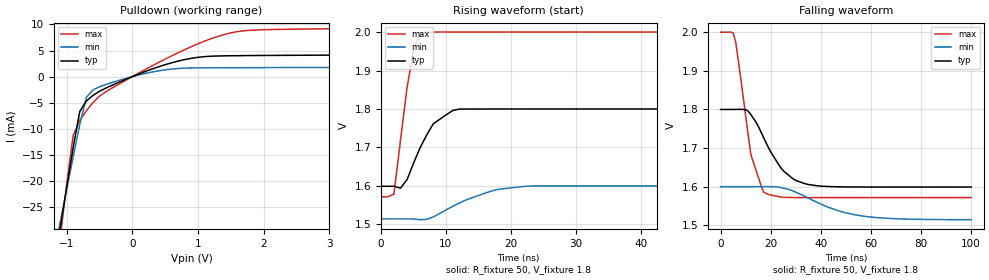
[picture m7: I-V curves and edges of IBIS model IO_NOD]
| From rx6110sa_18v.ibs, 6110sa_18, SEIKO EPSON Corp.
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[Model]   IO_NOD
Model_type Open_drain
Enable Active-Low
Polarity Non-Inverting
Vref=1.8
Vmeas=0.9
Rref=5000
C_comp   2.5p   2p   3p
[Temperature Range] 25   85   -40
[Voltage Range]   1.8   1.6   2.0
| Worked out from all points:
|   slope of the pulldown table from 0 to 0.27 V, typ, clamps not added: 206 ohm
|   falling waveform, R_fixture 50, V_fixture 1.8: 20-80 % time 10.6ns typ, 19.5ns min, 6.06ns max; typ from 1.8 V to 1.6 V
|   rising waveform, R_fixture 50, V_fixture 1.8: 20-80 % time 3.44ns typ, 6.96ns min, 2.06ns max; typ from 1.6 V to 1.8 V
[Pulldown]
-1.8V     -86.42mA   -77.23mA   -105.3mA
-1.1V     -29.16mA   -28.04mA   -31.08mA
-1V       -21.31mA   -21.63mA   -20.71mA
-900mV    -13.53mA   -15.35mA   -11.23mA
-800mV    -6.683mA   -9.177mA   -8.363mA
-700mV    -4.673mA   -3.993mA   -6.555mA
-500mV    -2.814mA   -1.945mA   -3.752mA
100mV     507uA      322.3uA    694.9uA
600mV     2.655mA    1.451mA    3.99mA
1.4V      3.983mA    1.706mA    8.072mA
1.9V      4.05mA     1.725mA    8.952mA
3.6V      4.155mA    1.772mA    9.24mA
[Falling Waveform]
R_fixture=50
V_fixture=1.8
V_fixture_min=1.6
V_fixture_max=2.0
0s        1.8V       1.6V       2V
5.051ns   1.8V       1.6V       1.998V
6.061ns   1.8V       1.6V       1.974V
10.1ns    1.799V     1.6V       1.78V
12.12ns   1.786V     1.6V       1.683V
17.17ns   1.727V     1.6V       1.586V
24.24ns   1.647V     1.597V     1.573V
34.34ns   1.607V     1.573V     1.572V
57.58ns   1.599V     1.523V     1.572V
100ns     1.599V     1.515V     1.572V
[Rising Waveform]
R_fixture=50
V_fixture=1.8
V_fixture_min=1.6
V_fixture_max=2.0
0s        1.599V     1.514V     1.572V
2.02ns    1.599V     1.514V     1.578V
3.03ns    1.594V     1.514V     1.718V
4.04ns    1.616V     1.514V     1.855V
5.051ns   1.659V     1.514V     1.953V
6.061ns   1.699V     1.512V     1.995V
7.071ns   1.732V     1.513V     1.999V
11.11ns   1.796V     1.547V     2V
22.22ns   1.8V       1.599V     2V
100ns     1.8V       1.6V       2V
[Ramp]
R_load=50
dV/dt_r   1.205E-1/3.396E-9   5.133E-2/6.953E-9   2.570E-1/2.043E-9
dV/dt_f   1.205E-1/1.061E-8   5.126E-2/1.954E-8   2.570E-1/6.054E-9
|[End   IO_NOD
